[IBIS ver]   3.2
[File name]   xio2000a.ibs
[File Rev]   1.0
[Date]   10/27/2010
[Source]   Data created at Wipro Technologies
[Notes]   Revision History:
   Rev 1.0: 08/05/2005
   Initial Model
   Rev 1.1: 10/27/2010
   Added model REFCLK for REFCLK- and REFCLK+
[Disclaimer] Please be aware that in the absence of a written agreement
   Texas Instruments(TI) assumes no liability for: (1) The
   accuracy of the IBIS models provided to your company (2) The
   proper functioning of these Models in your design or for any
   resulting applications;or (3) Infringement of
   patents,copyrights or intellectual property rights resulting
   from your use of these models. TI provides IBIS Models as a
   service to our customers and therefore reserves the right to
   limit distribution of the Models.
[Copyright]   Property of Texas Instruments Incorporated. Unauthorised
   reproduction and/or distribution is strictly prohibited. This
   product is protected under copyright law and trade secret law
   as an unpublished work. Created 1999,(C) Copyright 1999-2001,
   Texas Instruments Incorporated., All Rights Reserved. These
   commodities are under the U.S. Government distribution license
   control.As such,they are not to be re-exported without the
   prior approval of the U.S. Department of Commerce.
|   Component XIO2000A
[Component]   XIO2000
[Manufacturer]   Texas Instruments.
[Package]
| variable   typ   min   max
R_pkg   0.000   0.000   0.000
L_pkg   0.000H   0.000H   0.000H
C_pkg   0.000F   0.000F   0.000F
[Pin]  signal_name   model_name   R_pin   L_pin   C_pin
A10	GNT2#	UBT059	200.51m	3.0375n	0.34434p
A11	CLKOUT3	UBT059	197.19m	2.8806n	0.333p
A12	CLKOUT4	UBT059	206.46m	3.1016n	0.33795p
A13	CLKOUT5	UBT059	219m	3.3281n	0.38022p
A14	GNT5#	UBT059	233.41m	3.6498n	0.41982p
A15	EXT_ARB_EN	IC33SPD	246.26m	3.9009n	0.43852p
A16	REFCLK_SEL	IC33T	254.86m	4.1136n	0.43293p
A2	AD11	UBT059	257.13m	4.1211n	0.4061p
A3	AD9	UBT059	242.66m	3.8733n	0.44421p
A4	VCCP	Power	230.31m	3.5881n	0.42049p
A5	AD6	UBT059	218.12m	3.3291n	0.38752p
A6	AD4	UBT059	205.83m	3.1213n	0.34679p
A7	AD	UBT059	192.91m	2.7921n	0.35289p
A8	GNT0#	UBT059	187.24m	2.6487n	0.35797p
A9	GNT1#	UBT059	190.18m	2.7374n	0.36382p
B1	AD12	UBT059	259.07m	4.1327n	0.45318p
B10	CLKOUT2	UBT059	167.27m	2.3835n	0.38381p
B11	REQ3#	UBT059	176.07m	2.5991n	0.37177p
B12	REQ4#	UBT059	180.18m	2.5964n	0.3658p
B13	REQ5#	UBT059	191.25m	2.8154n	0.39873p
B14	CLKOUT6	UBT059	205.98m	3.2168n	0.42957p
B15	CLKRUN_EN	IC33SPD	214.26m	3.3165n	0.43973p
B17	VSSA	GND	258.7m	4.1403n	0.40885p
B3	AD10	UBT059	214.33m	3.2845n	0.45203p
B4	C/BE[0]#	UBT059	203.06m	3.1328n	0.42372p
B5	AD7	UBT059	189.2m	2.7673n	0.39683p
B6	AD5	UBT059	180.23m	2.6486n	0.36674p
B7	AD1	UBT059	172.49m	2.4897n	0.37825p
B8	REQ0#	UBT059	168.53m	2.4581n	0.37463p
B9	CLKOUT1	UBT059	167.15m	2.3971n	0.38272p
C1	AD14	UBT059	243.16m	3.8014n	0.46082p
C10	REQ2#	UBT059	145.16m	1.9646n	0.39508p
C11	GNT3#	UBT059	149.86m	2.0254n	0.34442p
C12	GNT4#	UBT059	154.19m	2.1146n	0.38133p
C13	VDD_33	Power	163.05m	2.2784n	0.41514p
C14	VSS	GND	178m	2.6389n	0.46221p
C16	REFCLK-	REFCLK	217.47m	3.354n	0.45738p
C17	REFCLK+	REFCLK	242.82m	3.8455n	0.44994p
C2	AD13	UBT059	217.31m	3.3174n	0.46908p
C4	AD8	UBT059	174.61m	2.5719n	0.45438p
C5	VSS	GND	161.71m	2.2854n	0.41066p
C6	VDD_33	Power	152.53m	2.0935n	0.37757p
C7	AD2	UBT059	148.98m	2.0036n	0.36538p
C8	CLKOUT0	UBT059	144.52m	1.9617n	0.36231p
C9	REQ1#	UBT059	143.24m	1.9385n	0.4173p
D1	C/BE[1]#	UBT059	231.87m	3.6059n	0.42434p
D10	VDD_33	Power	146.37m	1.8475n	0.4324p
D11	VSS	GND	151.67m	1.919n	0.54792p
D15	VDDA_33	Power	175.03m	2.5823n	0.45664p
D16	RSVD	Power	204.16m	3.1755n	0.42439p
D17	RSVD	IC33T	231.75m	3.6081n	0.39983p
D2	AD15	UBT059	204.08m	3.1367n	0.42517p
D3	VSS	GND	177.7m	2.6182n	0.45917p
D7	AD3	UBT059	150.6m	1.901n	0.4415p
D8	VSS	GND	144.13m	1.8192n	0.41812p
D9	VDD_15	Power	143.74m	1.8176n	0.42997p
E1	SERR#	UBT059	218.87m	3.337n	0.37776p
E15	VSSA	GND	147.99m	2.2908n	0.48818p
E16	RXN	EIO1G4A1W0_RXN	198.61m	2.8437n	0.49027p
E17	RXP	EIO1G4A1W0_RXP	197.04m	3.2043n	0.42236p
E2	PAR	UBT059	190.05m	2.7973n	0.40095p
E3	VDD_33	Power	163.49m	2.3364n	0.41638p
F1	DEVSEL#	UBT059	205.66m	3.1164n	0.33702p
F15	VSSA	GND	139.29m	2.0439n	0.48227p
F17	VDDA_15	Power	203.03m	2.8946n	0.33233p
F2	STOP#	UBT059	179.24m	2.5966n	0.36686p
F3	PERR#	UBT059	153.26m	2.1106n	0.38039p
G1	FRAME#	UBT059	196.03m	2.8783n	0.33248p
G14	VSSA	GND	157.79m	1.9609n	0.39948p
G15	VDDA_15	Power	148.97m	2.0029n	0.34662p
G17	VSS	GND	192.6m	2.8506n	0.34755p
G2	IRDY#	UBT059	173.46m	2.5324n	0.37009p
G3	TRDY#	UBT059	148.91m	2.0059n	0.33189p
G4	VSS	GND	150.38m	1.8964n	0.56408p
H1	C/BE[2]#	UBT059	200.52m	3.0501n	0.34251p
H14	VDD_15	Power	144.35m	1.8152n	0.3908p
H15	VSSA	GND	123.73m	1.8633n	0.48598p
H16	TXN	EIO1G4A1W0_TXN	174.36m	2.538n	0.47014p
H17	TXP	EIO1G4A1W0_TXP	176.76m	2.8196n	0.38129p
H2	AD17	UBT059	166.23m	2.3844n	0.38011p
H3	AD16	UBT059	143.93m	1.9491n	0.39407p
H4	VDD_33	Power	144.85m	1.8301n	0.2981p
J1	VCCP	Power	189.54m	2.7298n	0.36189p
J14	VDDA_15	Power	145m	1.8241n	0.41393p
J15	VDDA_15	Power	142.02m	1.9327n	0.36799p
J16	VSSA	GND	150.45m	2.3308n	0.40108p
J17	PERST#	IC33SFSHY	195.08m	2.9341n	0.37245p
J2	AD19	UBT059	166.79m	2.4214n	0.38316p
J3	AD18	UBT059	142.23m	1.9355n	0.41594p
J4	VDD_15	Power	142.59m	1.8047n	0.43204p
K1	AD20	UBT059	189.42m	2.7017n	0.36259p
K14	VDD_33_AUX	Power	144.8m	1.8281n	0.43281p
K15	VDDA_33	Power	143.51m	1.9496n	0.40034p
K16	VDD_33_COMB	Power	167.78m	2.4429n	0.38722p
K17	VSS	GND	200.3m	3.0279n	0.36505p
K2	AD21	UBT059	166.11m	2.3747n	0.37472p
K3	AD22	UBT059	143.96m	1.9513n	0.35242p
K4	VSS	GND	143.39m	1.8106n	0.41474p
L1	AD23	UBT059	191.77m	2.7588n	0.35421p
L14	VDD_33_COMBIO	Power	151.68m	1.9251n	0.55164p
L15	VSSA	GND	149.7m	2.0223n	0.33722p
L16	REF_PCIE	NC	173.15m	2.5232n	0.37883p
L17	REF1_PCIE	NC	196.26m	2.882n	0.33909p
L2	C/BE[3]#	UBT059	172.12m	2.4823n	0.3778p
L3	AD24	UBT059	148.94m	2.0056n	0.36648p
L4	AD25	UBT059	150.38m	1.9005n	0.43959p
M1	AD26	UBT059	207.8m	3.1781n	0.34798p
M15	PME#	IC33SFSHY	154.28m	2.1238n	0.37913p
M16	WAKE#	OUM42	180.26m	2.617n	0.36339p
M17	VDD_15_COMB	Power	206.41m	3.1046n	0.33365p
M2	AD27	UBT059	180.85m	2.6625n	0.36794p
M3	VDD_33	Power	153.11m	2.1117n	0.3791p
N1	AD28	UBT059	218.36m	3.3347n	0.37825p
N15	RSVD	IC33SHYPU	163.59m	2.3115n	0.41386p
N16	RSVD	IC33SHYPD	191.31m	2.8137n	0.40184p
N17	GRST#	IC33SHYPU	220.03m	3.3545n	0.3794p
N2	AD29	UBT059	190.68m	2.7994n	0.40166p
N3	VSS	GND	162.99m	2.3072n	0.41422p
P1	AD30	UBT059	231.57m	3.6105n	0.41403p
P10	VDD_33	Power	149.56m	1.8906n	0.42086p
P11	VDD_33	Power	162.95m	2.0539n	0.4636p
P15	VDD_15	Power	175.75m	2.5736n	0.46291p
P16	RSVD	NC	205.85m	3.185n	0.42913p
P17	RSVD	NC	232.73m	3.6099n	0.41756p
P2	AD31	UBT059	205.1m	3.1594n	0.42764p
P3	CLK	UBT059	176.74m	2.613n	0.45817p
P7	VDD_15	Power	146.81m	1.8583n	0.56787p
P8	VSS	GND	143.09m	1.8065n	0.43347p
P9	VDD_33	Power	144.27m	1.8236n	0.4424p
R1	M66EN	UBT059	243.49m	3.8412n	0.44561p
R10	VSS	GND	150.47m	2.02n	0.36427p
R11	VSS	GND	160.05m	2.1332n	0.39143p
R12	VSS	GND	169.77m	2.2596n	0.44803p
R13	VSS	GND	177.46m	2.4437n	0.32827p
R14	VDD_33	PHY1394	198.78m	2.8118n	0.96235p
R16	RSVD	NC	215.84m	3.2763n	0.45848p
R17	VSS	GND	244.18m	3.8908n	0.44792p
R2	INTA#	UBT059	216.57m	3.3037n	0.44088p
R4	VSS	GND	174.01m	2.5935n	0.46976p
R5	VDD_33	Power	159.73m	2.2568n	0.41857p
R6	VSS	GND	149.63m	2.0613n	0.38187p
R7	GPIO4_SCL	BC3350CTPU	146.24m	1.9761n	0.32888p
R8	RSVD	BC3350CS	142.67m	1.9354n	0.39819p
R9	RSVD	IC33T	144.75m	1.9581n	0.42919p
T1	INTB#	UBT059	258.28m	4.0927n	0.40644p
T10	RSVD	NC	173.53m	2.4939n	0.38119p
T11	RSVD	PHY1394	184.1m	2.6747n	0.40364p
T12	RSVD	PHY1394	193.93m	2.6651n	0.38639p
T13	VDD_33	Power	205.12m	2.9437n	0.44558p
T14	RSVD	PHY1394	227.87m	3.3807n	0.51943p
T15	RSVD	PHY1394	239.29m	3.5298n	0.52474p
T17	RSVD	NC	256.93m	4.1038n	0.43853p
T3	INTD#	UBT059	216.23m	3.2893n	0.47209p
T4	SERIRQ	UBT059	201.41m	3.1126n	0.43285p
T5	GPIO0_CLKRUN#	BC3350CTPU	186.79m	2.7427n	0.40379p
T6	GPIO2_INTEL_MODE	BC3350CTPU	177.38m	2.6194n	0.37136p
T7	GPIO5_SDA	BC3350CS	169.86m	2.4935n	0.37475p
T8	RSVD	BC3350CS	165.51m	2.3697n	0.38465p
T9	RSVD	IC33T	169.37m	2.4229n	0.39424p
U10	RSVD	IC33T	196.67m	2.8327n	0.3752p
U11	RSVD	PHY1394	202.22m	2.921n	0.37205p
U12	RSVD	PHY1394	216.2m	3.1024n	0.37714p
U13	RSVD	PHY1394	244.17m	3.6202n	0.41899p
U14	RSVD	PHY1394	248.69m	3.7543n	0.44792p
U15	RSVD	PHY1394	264.93m	4.0531n	0.64209p
U16	RSVD	PHY1394	280.63m	4.3306n	0.48279p
U2	INTC#	UBT059	258.33m	4.1239n	0.44959p
U3	PRST#	UBT059	240.48m	3.774n	0.32026p
U4	LOCK#	UBT059	228.47m	3.5904n	0.43151p
U5	GPIO1_PWR_OVER	BC3350CTPU	213.01m	3.2076n	0.389p
U6	GPIO3	BC3350CTPU	202.93m	3.082n	0.33684p
U7	GPIO6	BC3350CTPU	193.1m	2.8548n	0.33339p
U8	GPIO7	BC3350CTPU	198.34m	3.0217n	0.34819p
U9	RSVD	NC	191.45m	2.7869n	0.36729p
[Diff Pin]   inv_pin   vdiff   tdelay_typ
H16   H17   NA   NA
E16   E17   NA   NA
C17   C16   NA NA
[Model Selector]   BC3350BTPD
BC3350BTPD_2P5   Cell operated at VDDS=2.5V(typ) with Pulldown "on"
BC3350BTPDZ_2P5   Cell operated at VDDS=2.5V(typ) with Pulldown "off"
BC3350BTPD_3P3   Cell operated at VDDS=3.3V(typ) with Pulldown "on"
BC3350BTPDZ_3P3   Cell operated at VDDS=3.3V(typ) with Pulldown "off"
[Model Selector]   BC3350CS
BC3350CS_1P8   Cell operated at VDDS=1.8V(typ)
BC3350CS_2P5   Cell operated at VDDS=2.5V(typ)
BC3350CS_2P75   Cell operated at VDDS=2.75V(typ)
BC3350CS_3P3   Cell operated at VDDS=3.3V(typ)
[Model Selector]   BC3350CTPU
BC3350CTPU_2P5PU   Cell operated at VDDS=2.5V(typ) with Pulldown "on"
BC3350CTPU_2P5PUZ   Cell operated at VDDS=2.5V(typ) with Pulldown "off"
BC3350CTPU_3P3PU   Cell operated at VDDS=3.3V(typ) with Pulldown "on"
BC3350CTPU_3P3PUZ   Cell operated at VDDS=3.3V(typ) with Pulldown "off"
[Model Selector]   IC33SFSHY
IC33SFSHY_2P5   Cell operated at VDDS=2.5V(nom)
IC33SFSHY_3P3   Cell operated at VDDS=3.3V(nom)
[Model Selector]   IC33SHYPD
IC33SHYPD_2P5PD   Cell operated at VDDS=2.5V(typ)  with Pulldown "on"
IC33SHYPD_2P5PDZ   Cell operated at VDDS=2.5V(typ)  with Pulldown "off"
IC33SHYPD_2P75PD   Cell operated at VDDS=2.75V(typ) with Pulldown "on"
IC33SHYPD_2P75PDZ   Cell operated at VDDS=2.75V(typ) with Pulldown "off"
IC33SHYPD_3P3PD   Cell operated at VDDS=3.3V(typ)  with Pulldown "on"
IC33SHYPD_3P3PDZ   Cell operated at VDDS=3.3V(typ)  with Pulldown "off"
[Model Selector]   IC33SHYPU
IC33SHYPU_2P5PU   Cell operated at VDDS=2.5V(typ)  with Pullup "on"
IC33SHYPU_2P5PUZ   Cell operated at VDDS=2.5V(typ)  with Pullup "off"
IC33SHYPU_2P75PU   Cell operated at VDDS=2.75V(typ) with Pullup "on"
IC33SHYPU_2P75PUZ   Cell operated at VDDS=2.75V(typ) with Pullup "off"
IC33SHYPU_3P3PU   Cell operated at VDDS=3.3V(typ)  with Pullup "on"
IC33SHYPU_3P3PUZ   Cell operated at VDDS=3.3V(typ)  with Pullup "off"
[Model Selector]   IC33SPD
IC33SPD_2P5PD   Cell operated at VDDS=2.5V(typ) with pulldown "on"
IC33SPD_2P5PDZ   Cell operated at VDDS=2.5V(typ) with pulldown "off"
IC33SPD_3P3PD   Cell operated at VDDS=3.3V(typ) with pulldown "on"
IC33SPD_3P3PDZ   Cell operated at VDDS=3.3V(typ) with pulldown "off"
[Model Selector]   IC33T
IC33T_2P5   Cell operated at VDDS=2.5V(nom)
IC33T_3P3   Cell operated at VDDS=3.3V(nom)
[Model Selector]   OC3350BT
OC3350BT_2P5   Cell operated at VDDS=2.5V(nom)
OC3350BT_3P3   Cell operated at VDDS=3.3V(nom)
| Models and submodels in the file (42): BC3350BTPD_2P5 (I/O), BC3350BTPDZ_2P5 (I/O), BC3350BTPD_3P3 (I/O), BC3350BTPDZ_3P3 (I/O), BC3350CS_1P8 (I/O), BC3350CS_2P5 (I/O), BC3350CS_2P75 (I/O), BC3350CS_3P3 (I/O), BC3350CTPU_2P5PU (I/O), BC3350CTPU_2P5PUZ (I/O), BC3350CTPU_3P3PU (I/O), BC3350CTPU_3P3PUZ (I/O), EIO1G4A1W0_TXP (Output), EIO1G4A1W0_TXN (Output), EIO1G4A1W0_RXP (Input), EIO1G4A1W0_RXN (Input), IC33SFSHY_2P5 (Input), IC33SFSHY_3P3 (Input), IC33SHYPD_2P5PD (Input), IC33SHYPD_2P5PDZ (Input), IC33SHYPD_2P75PD (Input), IC33SHYPD_2P75PDZ (Input), IC33SHYPD_3P3PD (Input), IC33SHYPD_3P3PDZ (Input), IC33SHYPU_2P5PU (Input), IC33SHYPU_2P5PUZ (Input), IC33SHYPU_2P75PU (Input), IC33SHYPU_2P75PUZ (Input), IC33SHYPU_3P3PU (Input), IC33SHYPU_3P3PUZ (Input), IC33SPD_2P5PD (Input), IC33SPD_2P5PDZ (Input), IC33SPD_3P3PD (Input), IC33SPD_3P3PDZ (Input), IC33T_2P5 (Input), IC33T_3P3 (Input), OC3350BT_2P5 (3-state), OC3350BT_3P3 (3-state), OUM42 (Open_drain), PHY1394 (3-state), UBT059 (I/O), REFCLK (Input)
